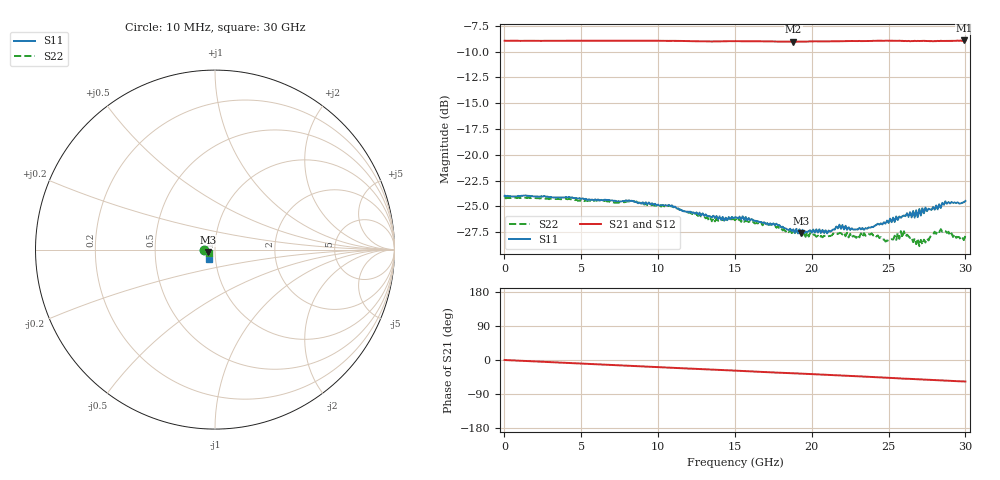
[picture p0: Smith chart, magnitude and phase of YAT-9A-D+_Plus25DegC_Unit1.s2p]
!Keysight Technologies,N5244A,MY52442000,A.10.40.14
!Model Number: YAT-9A-D+
!Date: Thursday, October 27, 2016 09:37:19
!Correction: S11(Full 2 Port(1,2))
!S21(Full 2 Port(1,2))
!S12(Full 2 Port(1,2))
!S22(Full 2 Port(1,2))
!S2P File: Measurements: S11, S21, S12, S22:
# Hz S  dB  R 50
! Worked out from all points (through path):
!   309 points, 10 MHz to 30 GHz, reference 50 ohm
!   highest |S21| = -8.93 dB at 29.9 GHz (marker M1); lowest = -9.1 dB at 18.8 GHz (marker M2)
!   group delay of S21, straight-line fit = 5.24 ps
!   lowest |S11| = -27.6 dB at 19.3 GHz (marker M3), VSWR 1.09, Z = 46.2 - j1.37 ohm
!   |S11| at or under -10 dB: start of sweep to end of sweep
!   |S22| runs from -28.8 to -24.1 dB; largest |S21 - S12| = 0.0045
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1e7  -23.97 -179.5  -8.96 0.2  -8.96 0.2  -24.15 -179.4
5.1e9  -24.22 -179.7  -8.96 -9.4  -8.97 -9.4  -24.43 177.5
1.01e10  -24.92 -178.4  -8.96 -19.0  -8.97 -18.8  -24.87 174.4
1.35e10  -26.04 -172.2  -9.03 -25.2  -9.03 -24.9  -26.43 176.9
1.51e10  -26.05 -170.1  -8.99 -28.2  -9.00 -27.9  -26.17 179.6
1.88e10  -27.22 -161.4  -9.05 -35.1  -9.05 -34.7  -27.25 -176.8
1.93e10  -27.61 -159.2  -9.04 -36.0  -9.03 -35.5  -27.55 -178.0
2.01e10  -27.24 -156.2  -9.02 -37.4  -9.01 -37.0  -27.72 -171.3
2.34e10  -27.28 -139.5  -8.98 -43.7  -9.01 -43.3  -27.58 -166.2
2.51e10  -26.18 -131.8  -8.95 -47.3  -8.96 -46.9  -28.28 -159.6
2.6e10  -25.87 -132.3  -8.98 -49.3  -9.00 -48.7  -27.40 -154.3
2.65e10  -26.06 -128.5  -8.98 -50.0  -8.99 -49.4  -27.96 -156.5
2.66e10  -25.44 -130.3  -8.99 -50.2  -8.98 -49.9  -28.45 -152.4
2.67e10  -26.08 -129.2  -8.96 -50.6  -8.97 -49.9  -28.08 -155.1
2.68e10  -25.37 -130.1  -8.98 -50.8  -8.99 -50.3  -28.64 -153.7
2.69e10  -26.04 -129.9  -8.97 -51.0  -8.98 -50.3  -28.10 -154.7
2.7e10  -25.25 -128.7  -8.98 -51.1  -8.99 -50.7  -28.84 -155.6
2.71e10  -25.88 -130.2  -8.97 -51.4  -8.99 -50.8  -28.24 -154.5
2.72e10  -25.17 -127.0  -8.96 -51.4  -8.99 -51.2  -28.68 -156.3
2.84e10  -25.15 -128.2  -8.96 -53.8  -8.99 -53.2  -27.21 -154.3
2.99e10  -24.59 -122.9  -8.93 -56.7  -8.98 -56.2  -28.25 -148.3
3e10  -24.46 -122.9  -8.94 -56.8  -8.94 -56.5  -27.82 -150.3
